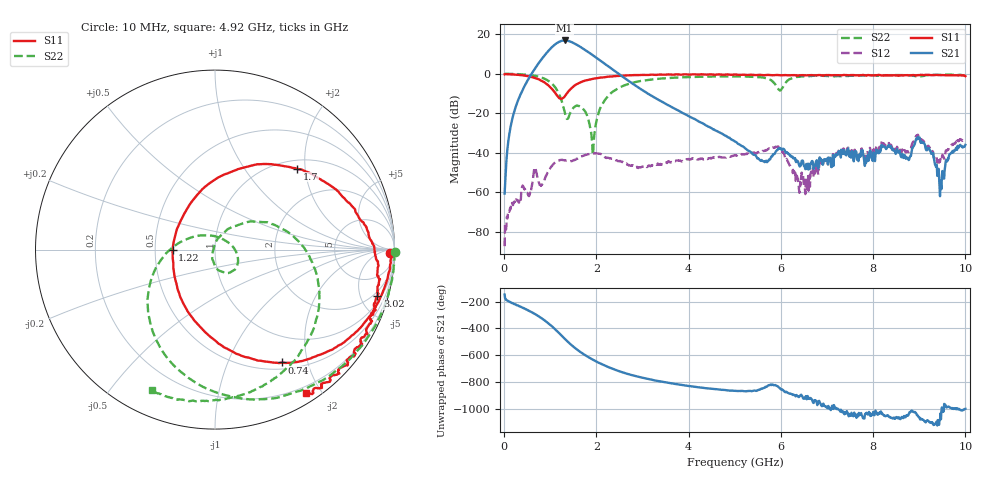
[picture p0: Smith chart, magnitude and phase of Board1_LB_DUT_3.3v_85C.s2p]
! Created Tue May 27 16:26:43 2025
# hz S ma R 50
! 2 Port Network Data from SP1.SP block
! freq  magS11  angS11  magS21  angS21  magS12  angS12  magS22  angS22
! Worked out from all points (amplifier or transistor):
!   1000 points, 10 MHz to 10 GHz, reference 50 ohm
!   highest |S21| = 17.0 dB at 1.31 GHz (marker M1)
!   |S21| within 3 dB of that: 1.054 GHz to 1.635 GHz (581.1 MHz wide, 43.2 % of centre)
!   unconditionally stable (mu >= 1): 58.46 MHz to 62.7 MHz; 89.92 MHz to 103.8 MHz; 115.6 MHz to end of sweep
!   at 1.67 GHz: K = 8.19, MAG = 15.6 dB, |S12| = -42.0 dB
!   at 5.01 GHz: K = 47.54, MAG = -16.3 dB, |S12| = -41.3 dB
!   at 10 GHz: K = 55.57, MAG = -21.9 dB, |S12| = -33.1 dB
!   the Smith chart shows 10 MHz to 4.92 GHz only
!   S11 on the Smith chart (normalised r, x): 10 MHz: 53, -35; 740 MHz: 0.59, -1.60; 1.22 GHz: 0.62, -0.00; 1.7 GHz: 1.18, +1.81; 3.02 GHz: 1.47, -6.77; 4.92 GHz: 0.12, -1.81
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1e7  0.9742 -1.0  0.0009186 -146.7  4.249e-05 21.7  1.005 -0.8
2.1e8  0.964 -14.4  0.1017 144.5  0.0005334 74.4  0.9954 -18.7
7.4e8  0.7316 -59.3  1.805 52.4  0.001942 59.4  0.8559 -77.1
9e8  0.579 -79.9  3.183 14.4  0.002519 110.4  0.7293 -101.8
1.04e9  0.4105 -106.5  4.818 -25.0  0.004659 100.8  0.5589 -129.3
1.13e9  0.3033 -133.5  5.911 -53.7  0.00596 86.2  0.4151 -151.3
1.22e9  0.2363 -179.5  6.725 -84.5  0.006549 71.3  0.2526 -179.5
1.31e9  0.2648 129.7  7.051 -115.7  0.006475 60.2  0.1108 134.2
1.47e9  0.4436 78.0  6.354 -167.1  0.006123 56.5  0.1224 -9.9
1.68e9  0.6272 46.5  4.617 137.8  0.008016 49.6  0.1417 -65.8
1.7e9  0.6425 44.6  4.465 133.2  0.008217 48.3  0.133 -70.2
1.9e9  0.741 28.1  3.108 91.4  0.009416 29.9  0.02268 -127.6
2.11e9  0.812 16.0  2.082 54.1  0.009151 6.1  0.1553 53.5
2.48e9  0.888 0.1  1.007 2.2  0.006082 -5.1  0.437 10.5
3.02e9  0.9415 -16.1  0.3724 -49.8  0.004411 6.3  0.677 -32.5
3.34e9  0.952 -24.4  0.2214 -72.7  0.00508 8.0  0.7499 -51.4
4.92e9  0.9474 -57.7  0.02207 -144.0  0.008054 -6.9  0.8597 -114.3
5.01e9  0.9683 -59.6  0.01914 -145.7  0.008634 -10.5  0.8624 -117.7
6.67e9  0.9313 -90.9  0.00611 149.6  0.004008 145.7  0.8868 -149.6
8.34e9  0.9118 -135.8  0.0159 21.1  0.01766 31.6  0.9194 172.8
9.49e9  0.9303 -167.9  0.002413 90.1  0.007434 67.4  0.9532 164.3
1e10  0.8763 177.8  0.01582 79.8  0.02222 72.1  0.9133 163.4
